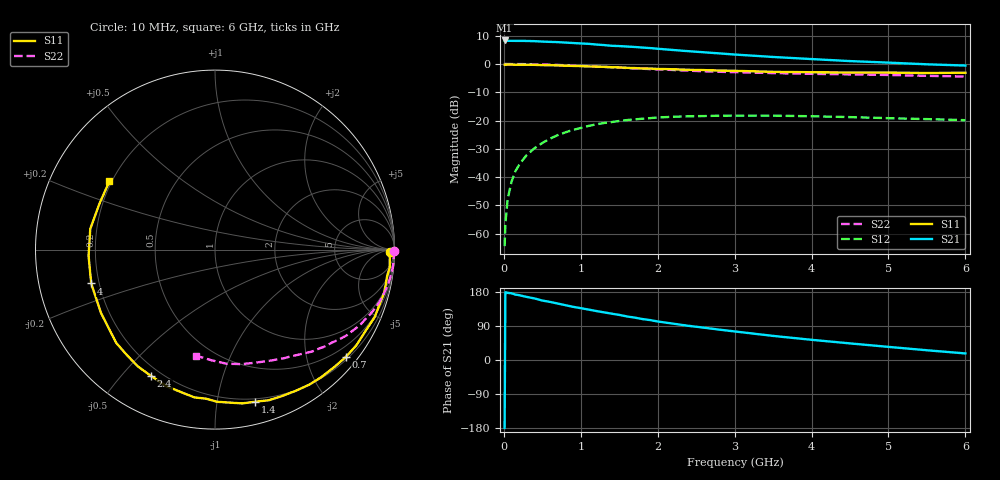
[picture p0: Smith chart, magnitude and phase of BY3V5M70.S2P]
! SIEMENS Small Signal Semiconductors
! BFY420
! Si NPN RF SIEGET Grounded Emitter Transistor in MICRO-X
! VCE = 3.5 V  IC = 0.7 mA
! Common Emitter S-Parameters:  October  1996
# GHz  S  MA  R  50
!  f  S11  S21  S12  S22
! GHz  MAG  ANG  MAG  ANG  MAG  ANG  MAG  ANG
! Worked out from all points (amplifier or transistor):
!   36 points, 10 MHz to 6 GHz, reference 50 ohm
!   highest |S21| = 8.3 dB at 10 MHz (marker M1)
!   |S21| within 3 dB of that: start of sweep to 2.032 GHz
!   unconditionally stable (mu >= 1): 4.648 GHz to end of sweep
!   at 250 MHz: K = 0.02, MSG = 21.0 dB, |S12| = -33.8 dB
!   at 1.4 GHz: K = 0.16, MSG = 13.5 dB, |S12| = -20.6 dB
!   at 6 GHz: K = 1.40, MAG = 5.9 dB, |S12| = -19.9 dB
!   S11 on the Smith chart (normalised r, x): 10 MHz: 59, -31; 700 MHz: 0.26, -2.77; 1.4 GHz: 0.18, -1.29; 2.4 GHz: 0.16, -0.60; 4 GHz: 0.17, -0.13; 6 GHz: 0.19, +0.29
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0.01  0.9739 -0.8  2.607 -179.3  0.0006 91.6  0.9989 -0.3
0.02  0.9702 -1.3  2.601 178.8  0.0015 76.1  0.9999 -0.5
0.05  0.9753 -2.8  2.569 177.2  0.0041 88.2  0.9986 -1.3
0.1  0.9783 -6.0  2.568 176.0  0.0083 85.2  0.9965 -2.6
0.15  0.9706 -8.5  2.563 172.6  0.0127 82.4  0.9961 -4.0
0.3  0.968 -16.9  2.552 166.3  0.0248 79.3  0.9915 -7.7
0.4  0.966 -22.9  2.534 162.4  0.0325 76.0  0.9858 -10.3
0.5  0.9532 -28.5  2.49 156.9  0.0401 73.1  0.9787 -12.8
0.7  0.9428 -39.4  2.436 149.0  0.0552 66.2  0.9612 -17.7
0.9  0.9249 -50.2  2.349 140.3  0.0683 59.2  0.9378 -22.4
1.1  0.9061 -60.4  2.273 133.1  0.0802 53.3  0.9135 -26.9
1.4  0.8769 -75.1  2.098 122.3  0.0938 44.9  0.8765 -32.9
1.6  0.8555 -84.9  2.036 114.9  0.1019 39.5  0.847 -36.7
1.8  0.8321 -93.5  1.952 108.1  0.1076 34.7  0.8237 -40.0
2.2  0.8072 -109.7  1.768 96.0  0.1166 25.9  0.7837 -46.5
2.4  0.7892 -116.8  1.684 90.2  0.1189 22.4  0.7609 -49.5
2.8  0.7656 -129.9  1.539 80.1  0.1217 15.7  0.7277 -55.0
3.5  0.7266 -151.0  1.331 63.6  0.122 7.0  0.6903 -63.8
4  0.715 -164.7  1.222 53.3  0.119 2.2  0.6696 -70.1
4.5  0.7053 -177.2  1.125 43.8  0.115 -1.6  0.6555 -76.7
5.5  0.6928 158.3  0.987 25.7  0.106 -4.1  0.6173 -91.7
6  0.7008 147.1  0.938 17.3  0.1015 -3.0  0.6004 -100.1
